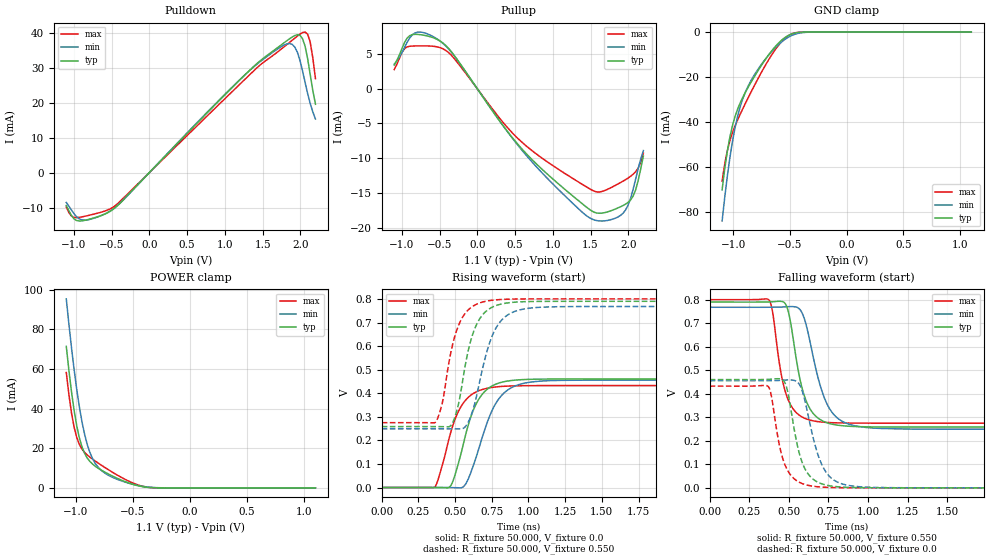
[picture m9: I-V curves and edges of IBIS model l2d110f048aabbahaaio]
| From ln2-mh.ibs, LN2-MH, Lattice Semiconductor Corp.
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|   Model l2d110f048aabbahaaio
[Model] l2d110f048aabbahaaio
| Clamp models do not include dynamic input termination. Please refer to
| the l2d110axxxaabbahaain model for input termination.
Model_type I/O
Polarity   Non-Inverting
Enable   Active-Low
Vinl =  0.200V
Vinh =  0.300V
Vmeas =  0.550V
Cref =  20.000pF
Rref =  50.000
Vref =  0.600V
C_comp   2.000pF   1.500pF   2.500pF
[Temperature Range]   25.000   0.125k   -40.000
[Voltage Range]   1.100V   1.070V   1.130V
[C Comp Corner]
C_comp   2.000pF   1.500pF   2.500pF
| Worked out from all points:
|   slope of the pulldown table from 0 to 0.165 V, typ, clamps not added: 44.4 ohm
|   slope of the pullup table from 0 to 0.165 V, typ, clamps not added: 63.1 ohm
|   GND clamp passes 1 mA (typ) near -0.49 V on its own axis
|   POWER clamp passes 1 mA (typ) near -0.45 V on its own axis
|   rising waveform, R_fixture 50.000, V_fixture 0.0: 20-80 % time 138ps typ, 162ps min, 134ps max; typ from 0 V to 0.461 V
|   rising waveform, R_fixture 50.000, V_fixture 0.550: 20-80 % time 114ps typ, 135ps min, 109ps max; typ from 0.259 V to 0.791 V
|   falling waveform, R_fixture 50.000, V_fixture 0.550: 20-80 % time 96.4ps typ, 124ps min, 84ps max; typ from 0.791 V to 0.259 V
|   falling waveform, R_fixture 50.000, V_fixture 0.0: 20-80 % time 89.6ps typ, 110ps min, 82.2ps max; typ from 0.461 V to 0 V
[Pulldown]
|Voltage   I(typ)   I(min)   I(max)
-1.1V     -9.41mA    -8.535mA   -9.849mA
-1.032V   -12.26mA   -10.69mA   -12.43mA
-896mV    -13.83mA   -13.52mA   -12.69mA
-488mV    -10.64mA   -10.58mA   -10.02mA
1.246V    27.54mA    27.59mA    26.3mA
1.824V    37.8mA     36.87mA    36.7mA
1.926V    39.24mA    35.96mA    38.49mA
1.96V     39.48mA    34.49mA    39.08mA
2.028V    38.4mA     29.21mA    40.09mA
2.096V    32.66mA    22.68mA    39.63mA
2.13V     28.15mA    19.83mA    37.42mA
2.2V      19.56mA    15.36mA    26.91mA
[Pullup]
|Voltage   I(typ)   I(min)   I(max)
-1.1V     3.391mA    3.517mA    2.749mA
-996mV    5.814mA    5.23mA     5.224mA
-894mV    7.622mA    7.298mA    6.097mA
-758mV    7.769mA    8.144mA    6.15mA
-486mV    6.803mA    6.791mA    5.876mA
-316mV    4.941mA    4.892mA    4.481mA
568mV     -8.372mA   -8.524mA   -7.458mA
1.554V    -17.78mA   -18.88mA   -14.76mA
1.792V    -17.46mA   -18.76mA   -14.11mA
1.962V    -16.61mA   -17.47mA   -13.09mA
2.098V    -14.53mA   -12.98mA   -11.92mA
2.2V      -9.694mA   -8.899mA   -9.266mA
[GND_clamp]
|Voltage   I(typ)   I(min)   I(max)
-1.1V     -70.17mA   -84.03mA   -66.26mA
-1.054V   -53mA      -64.11mA   -52.77mA
-1.008V   -41.47mA   -48.47mA   -44.67mA
-962mV    -34.12mA   -37.21mA   -38.94mA
-916mV    -28.89mA   -29.48mA   -33.96mA
-847mV    -22.51mA   -21.78mA   -26.94mA
-778mV    -16.78mA   -16.17mA   -20.25mA
-663mV    -8.428mA   -8.708mA   -10.22mA
-571mV    -3.466mA   -4.237mA   -4.093mA
-502mV    -1.18mA    -1.941mA   -1.256mA
-410mV    -105.5uA   -402.4uA   -63.37uA
1.1V      0A         0A         0A
[POWER_clamp]
|Voltage   I(typ)   I(min)   I(max)
-1.085V   71.41mA    95.35mA    58.18mA
-1.062V   59.23mA    82.55mA    46.99mA
-1.039V   48.36mA    70.56mA    37.71mA
-1.016V   38.97mA    59.53mA    30.53mA
-970mV    25.17mA    40.76mA    21.88mA
-924mV    17.37mA    26.93mA    17.87mA
-901mV    15.03mA    21.86mA    16.59mA
-855mV    12.01mA    14.79mA    14.5mA
-763mV    8.448mA    8.108mA    10.89mA
-533mV    2.369mA    2.267mA    3.272mA
-349mV    143.9uA    291.4uA    171.3uA
1.1V      0A         0A         0A
[Ramp]
| variable   typ   min   max
dV/dt_r   0.277/0.138n   0.274/0.162n   0.260/0.134n
dV/dt_f   0.349/0.106n   0.341/0.142n   0.349/87.474p
R_load = 50.000
[Rising Waveform]
R_fixture= 50.000
V_fixture= 0.0
V_fixture_min= 0.0
V_fixture_max= 0.0
|time   V(typ)   V(min)   V(max)
0s        1.208uV    6.471uV    552nV
361ps     77.98uV    49.82uV    2.025mV
470ps     7.783mV    -243.9uV   233.5mV
557ps     186.8mV    3.843mV    359.7mV
619ps     320.7mV    84.28mV    397.5mV
689ps     399.3mV    221.2mV    417.1mV
795ps     443.2mV    374.2mV    428.4mV
934ps     457.5mV    437.2mV    432.3mV
1.406ns   461.1mV    456.2mV    433.2mV
10ns      461.1mV    456.3mV    433.1mV
[Rising Waveform]
R_fixture= 50.000
V_fixture= 0.550
V_fixture_min= 0.534
V_fixture_max= 0.568
|time   V(typ)   V(min)   V(max)
0s        258.9mV    249.5mV    275.5mV
370ps     259mV      249.5mV    280.4mV
414ps     258.5mV    249.5mV    363.3mV
484ps     276.5mV    249.1mV    610.1mV
566ps     507.8mV    256.2mV    737.8mV
649ps     696.1mV    396.5mV    779.8mV
783ps     774.1mV    682.6mV    797.7mV
921ps     788.2mV    751.3mV    801mV
1.199ns   791.2mV    768.4mV    801.6mV
10ns      791.2mV    769.2mV    801.6mV
[Falling Waveform]
R_fixture= 50.000
V_fixture= 0.550
V_fixture_min= 0.534
V_fixture_max= 0.568
|time   V(typ)   V(min)   V(max)
0s        791.2mV    769.2mV    801.6mV
376ps     791.7mV    769.2mV    798.5mV
398ps     792.5mV    769.3mV    745.7mV
475ps     786.3mV    770.8mV    415.5mV
504ps     728.8mV    771.9mV    362.5mV
596ps     395mV      723.8mV    297.5mV
724ps     281.4mV    383.1mV    279.3mV
865ps     263mV      274.5mV    276.1mV
1.219ns   259mV      250.7mV    275.5mV
10ns      258.9mV    249.5mV    275.5mV
[Falling Waveform]
R_fixture= 50.000
V_fixture= 0.0
V_fixture_min= 0.0
V_fixture_max= 0.0
|time   V(typ)   V(min)   V(max)
0s        461.1mV    456.3mV    433.1mV
370ps     461.9mV    456.3mV    431.2mV
390ps     462.8mV    456.5mV    389.7mV
442ps     464.2mV    457.6mV    176.1mV
478ps     443.1mV    459mV      93.92mV
553ps     182.7mV    451.2mV    28.68mV
613ps     67.54mV    336mV      12.02mV
697ps     19.69mV    116.4mV    3.786mV
824ps     3.792mV    19.43mV    708.6uV
10ns      1.208uV    6.462uV    556.6nV
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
